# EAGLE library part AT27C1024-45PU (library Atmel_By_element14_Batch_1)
1-Megabit OTP EPROM
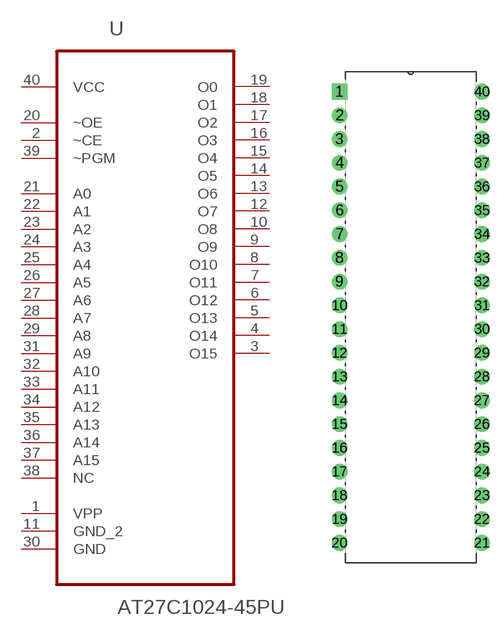
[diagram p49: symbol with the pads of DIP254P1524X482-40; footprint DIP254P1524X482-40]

Designator prefix U

## AT27C1024-45PU (DESCRIPTION: 1-Megabit OTP EPROM; MPN: AT27C1024-45PU; OC_FARNELL: 1841587; OC_NEWARK: 12T1363; PACKAGE: DIP-40; SUPPLIER: Atmel)  [DIP254P1524X482-40]
1  VPP  pwr
2  ~CE  in
3  O15  out
4  O14  out
5  O13  out
6  O12  out
7  O11  out
8  O10  out
9  O9  out
10  O8  out
11  GND_2  pas
12  O7  out
13  O6  out
14  O5  out
15  O4  out
16  O3  out
17  O2  out
18  O1  out
19  O0  out
20  ~OE  in
21  A0  in
22  A1  in
23  A2  in
24  A3  in
25  A4  in
26  A5  in
27  A6  in
28  A7  in
29  A8  in
30  GND  pas
31  A9  in
32  A10  in
33  A11  in
34  A12  in
35  A13  in
36  A14  in
37  A15  in
38  NC  nc
39  ~PGM  in
40  VCC  pwr

## Footprint DIP254P1524X482-40 (pad centres in mm)
drill 1.118 square: 1 -15.24,48.26
drill 1.118: 2 -15.24,45.72; 3 -15.24,43.18; 4 -15.24,40.64; 5 -15.24,38.1; 6 -15.24,35.56; 7 -15.24,33.02; 8 -15.24,30.48; 9 -15.24,27.94; 10 -15.24,25.4; 11 -15.24,22.86; 12 -15.24,20.32; 13 -15.24,17.78; 14 -15.24,15.24; 15 -15.24,12.7; 16 -15.24,10.16; 17 -15.24,7.62; 18 -15.24,5.08; 19 -15.24,2.54; 20 -15.24,0; 21 0,0; 22 0,2.54; 23 0,5.08; 24 0,7.62; 25 0,10.16; 26 0,12.7; 27 0,15.24; 28 0,17.78; 29 0,20.32; 30 0,22.86; 31 0,25.4; 32 0,27.94; 33 0,30.48; 34 0,33.02; 35 0,35.56; 36 0,38.1; 37 0,40.64; 38 0,43.18; 39 0,45.72; 40 0,48.26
